| TEXAS INSTRUMENTS INCORPORATED
| Standard Linear and Logic Group
| IBIS Model of SN74LVCZ16245A
| 16-BIT BUS TRANSCEIVER WITH 3-STATE OUTPUTS
| This file contains package information for the following:
|  TSSOP 48-pin (DGG) package as [Component] LVCZ16245A_DGG
|  TVSOP 48-pin (DGV) package as [Component] LVCZ16245A_DGV
|  SSOP 48-pin (DL) package as [Component] LVCZ16245A_DL
| This device can be powered at the following Vccs:
|  2.7 volt Vcc
|  3.3 volt Vcc
| This file provides unique models under the [Model Selector] for each Vcc.
| For operation at a specific Vcc, select the appropriate model after each
| [Model Selector] keyword.
[IBIS Ver]   3.2
[Comment char]  |_char
[File Name]   sn74lvcz16245a.ibs
[File Rev]   1.1 | x_die
[Date]   March 01,2004
[Source]   Data created from TI-SPICE simulations at TI-SLL.
[Notes]   The following is an IBIS list for the LVCZ16245A.
   Please contact sllibis@ti.com with questions and
   comments concerning SLL IBIS models.
   - FILE REV HISTORY
   - 1.1 Release IBIS file on 03/02/04
   - Power clamp data deleted as there is no power-clamp diode.
[Disclaimer] Property of Texas Instruments Incorporated.  Unauthorized
   reproduction and/or distribution is strictly prohibited.
   This product is protected under copyright law.
   Created  2004, (C) Copyright  2004, Texas Instruments
   Incorporated, All Rights Reserved
   UNLESS THERE IS A SIGNED, WRITTEN AGREEMENT TO THE
   CONTRARY, TEXAS INSTRUMENTS (TI) IS PROVIDING THE IBIS
   MODELS  AND WITHOUT ANY WARRANTY, EXPRESSED OR
   IMPLIED.  TI assumes no liability for:
   1) the accuracy of the IBIS models provided to your
   company;
   2) the proper functioning of these IBIS Models in your
   design or for any resulting applications; or
   3) infringement of patents, copyrights or intellectual
   property rights resulting from your use of these IBIS
   models.
   TI provides IBIS Models as a service to our customers.
   You and your company shall not distribute, sell or give
   these models to anyone else without prior written
   permission from TI.
   TI reserves the right to make changes to our products or
   to discontinue any semiconductor product or service
   without notice, and advises our customers to obtain the
   latest version of relevant information to verify, before
   placing orders, that the information being relied on is
   current.
   Please be aware that your receipt and use of the IBIS
   information provided shall serve as acceptance of these
   terms and conditions.  If you do not accept these terms,
   you should return or destroy the IBIS models and any
   other accompanying information immediately.
| Component LVCZ16245A_DGG 48-pin TSSOP
[Component]   LVCZ16245A_DGG
[Manufacturer]   Texas Instruments, Inc.
[Package]
|   typ   min   max
R_pkg   4.400e-02   3.800e-02   5.100e-02
L_pkg   3.019e-09   2.486e-09   4.099e-09
C_pkg   5.070e-13   3.340e-13   8.090e-13
[Pin]   signal_name   model_name   R_pin   L_pin   C_pin
1   1DIR   LVCZ16245A_DIR   4.100e-02   4.017e-09   7.590e-13
2   1B1   LVCZ16245A_IO   4.200e-02   3.737e-09   7.920e-13
3   1B2   LVCZ16245A_IO   4.200e-02   3.480e-09   6.610e-13
4   GND   GND   3.800e-02   3.131e-09   5.750e-13
5   1B3   LVCZ16245A_IO   4.700e-02   3.122e-09   5.660e-13
6   1B4   LVCZ16245A_IO   4.300e-02   2.948e-09   5.040e-13
7   VCC   POWER   4.500e-02   2.845e-09   3.970e-13
8   1B5   LVCZ16245A_IO   4.900e-02   2.835e-09   3.940e-13
9   1B6   LVCZ16245A_IO   4.800e-02   2.715e-09   3.780e-13
10   GND   GND   5.000e-02   2.664e-09   3.630e-13
11   1B7   LVCZ16245A_IO   5.000e-02   2.585e-09   3.480e-13
12   1B8   LVCZ16245A_IO   4.900e-02   2.550e-09   3.370e-13
13   2B1   LVCZ16245A_IO   4.900e-02   2.541e-09   3.360e-13
14   2B2   LVCZ16245A_IO   5.000e-02   2.574e-09   3.480e-13
15   GND   GND   4.900e-02   2.618e-09   3.590e-13
16   2B3   LVCZ16245A_IO   4.600e-02   2.671e-09   3.750e-13
17   2B4   LVCZ16245A_IO   4.500e-02   2.754e-09   3.890e-13
18   VCC   POWER   4.400e-02   2.823e-09   4.500e-13
19   2B5   LVCZ16245A_IO   4.200e-02   2.968e-09   5.030e-13
20   2B6   LVCZ16245A_IO   5.100e-02   3.108e-09   5.350e-13
21   GND   GND   4.200e-02   3.175e-09   5.870e-13
22   2B7   LVCZ16245A_IO   4.100e-02   3.449e-09   6.780e-13
23   2B8   LVCZ16245A_IO   4.400e-02   3.766e-09   8.040e-13
24   2DIR   LVCZ16245A_DIR   4.300e-02   4.065e-09   7.610e-13
25   2OE   LVCZ16245A_NOE   4.100e-02   3.994e-09   7.570e-13
26   2A8   LVCZ16245A_IO   3.900e-02   3.649e-09   7.890e-13
27   2A7   LVCZ16245A_IO   3.800e-02   3.362e-09   6.600e-13
28   GND   GND   3.800e-02   3.082e-09   5.740e-13
29   2A6   LVCZ16245A_IO   4.400e-02   2.990e-09   5.220e-13
30   2A5   LVCZ16245A_IO   4.100e-02   2.917e-09   4.950e-13
31   VCC   POWER   4.300e-02   2.820e-09   4.480e-13
32   2A4   LVCZ16245A_IO   4.300e-02   2.699e-09   3.850e-13
33   2A3   LVCZ16245A_IO   4.500e-02   2.628e-09   3.720e-13
34   GND   GND   4.600e-02   2.556e-09   3.560e-13
35   2A2   LVCZ16245A_IO   4.600e-02   2.495e-09   3.440e-13
36   2A1   LVCZ16245A_IO   4.700e-02   2.487e-09   3.340e-13
37   1A8   LVCZ16245A_IO   4.700e-02   2.490e-09   3.350e-13
38   1A7   LVCZ16245A_IO   4.600e-02   2.486e-09   3.430e-13
39   GND   GND   4.500e-02   2.566e-09   3.560e-13
40   1A6   LVCZ16245A_IO   4.400e-02   2.639e-09   3.740e-13
41   1A5   LVCZ16245A_IO   4.300e-02   2.701e-09   3.860e-13
42   VCC   POWER   4.300e-02   2.817e-09   4.500e-13
43   1A4   LVCZ16245A_IO   4.100e-02   2.935e-09   5.010e-13
44   1A3   LVCZ16245A_IO   4.700e-02   3.035e-09   5.290e-13
45   GND   GND   4.300e-02   3.171e-09   5.890e-13
46   1A2   LVCZ16245A_IO   4.000e-02   3.415e-09   6.820e-13
47   1A1   LVCZ16245A_IO   4.300e-02   3.741e-09   8.090e-13
48   1OE   LVCZ16245A_NOE   4.400e-02   4.099e-09   7.640e-13
| Component LVCZ16245A_DGV 48-pin TVSOP
[Component]   LVCZ16245A_DGV
[Manufacturer]   Texas Instruments, Inc.
[Package]
|   typ   min   max
R_pkg   7.000e-02   4.900e-02   8.500e-02
L_pkg   3.013e-09   2.743e-09   3.408e-09
C_pkg   3.710e-13   2.940e-13   5.110e-13
[Pin]   signal_name   model_name   R_pin   L_pin   C_pin
1   1DIR   LVCZ16245A_DIR   4.900e-02   3.393e-09   4.970e-13
2   1B1   LVCZ16245A_IO   6.000e-02   3.250e-09   5.020e-13
3   1B2   LVCZ16245A_IO   7.700e-02   3.310e-09   4.510e-13
4   GND   GND   8.500e-02   3.299e-09   4.040e-13
5   1B3   LVCZ16245A_IO   8.300e-02   3.136e-09   3.600e-13
6   1B4   LVCZ16245A_IO   7.700e-02   3.019e-09   3.630e-13
7   VCC   POWER   6.500e-02   2.882e-09   3.490e-13
8   1B5   LVCZ16245A_IO   6.600e-02   2.829e-09   3.140e-13
9   1B6   LVCZ16245A_IO   6.700e-02   2.796e-09   3.140e-13
10   GND   GND   6.900e-02   2.754e-09   3.080e-13
11   1B7   LVCZ16245A_IO   7.000e-02   2.753e-09   3.010e-13
12   1B8   LVCZ16245A_IO   7.100e-02   2.745e-09   2.940e-13
13   2B1   LVCZ16245A_IO   7.000e-02   2.744e-09   2.940e-13
14   2B2   LVCZ16245A_IO   7.000e-02   2.754e-09   3.010e-13
15   GND   GND   6.900e-02   2.754e-09   3.080e-13
16   2B3   LVCZ16245A_IO   6.700e-02   2.796e-09   3.140e-13
17   2B4   LVCZ16245A_IO   6.600e-02   2.829e-09   3.140e-13
18   VCC   POWER   6.500e-02   2.883e-09   3.500e-13
19   2B5   LVCZ16245A_IO   7.500e-02   3.014e-09   3.630e-13
20   2B6   LVCZ16245A_IO   8.000e-02   3.128e-09   3.580e-13
21   GND   GND   8.400e-02   3.295e-09   4.030e-13
22   2B7   LVCZ16245A_IO   7.800e-02   3.311e-09   4.520e-13
23   2B8   LVCZ16245A_IO   6.200e-02   3.259e-09   5.010e-13
24   2DIR   LVCZ16245A_DIR   5.200e-02   3.404e-09   4.960e-13
25   2OE   LVCZ16245A_NOE   5.300e-02   3.397e-09   5.050e-13
26   2A8   LVCZ16245A_IO   6.200e-02   3.249e-09   5.110e-13
27   2A7   LVCZ16245A_IO   7.700e-02   3.308e-09   4.530e-13
28   GND   GND   8.200e-02   3.289e-09   4.030e-13
29   2A6   LVCZ16245A_IO   7.800e-02   3.121e-09   3.590e-13
30   2A5   LVCZ16245A_IO   7.400e-02   3.010e-09   3.630e-13
31   VCC   POWER   6.500e-02   2.883e-09   3.490e-13
32   2A4   LVCZ16245A_IO   6.700e-02   2.829e-09   3.140e-13
33   2A3   LVCZ16245A_IO   6.700e-02   2.795e-09   3.140e-13
34   GND   GND   6.900e-02   2.753e-09   3.070e-13
35   2A2   LVCZ16245A_IO   7.000e-02   2.753e-09   3.010e-13
36   2A1   LVCZ16245A_IO   7.000e-02   2.743e-09   2.940e-13
37   1A8   LVCZ16245A_IO   7.000e-02   2.743e-09   2.940e-13
38   1A7   LVCZ16245A_IO   7.000e-02   2.753e-09   3.010e-13
39   GND   GND   6.900e-02   2.754e-09   3.070e-13
40   1A6   LVCZ16245A_IO   6.800e-02   2.797e-09   3.140e-13
41   1A5   LVCZ16245A_IO   6.700e-02   2.830e-09   3.140e-13
42   VCC   POWER   6.400e-02   2.880e-09   3.490e-13
43   1A4   LVCZ16245A_IO   7.200e-02   3.004e-09   3.620e-13
44   1A3   LVCZ16245A_IO   7.800e-02   3.121e-09   3.590e-13
45   GND   GND   8.400e-02   3.296e-09   4.030e-13
46   1A2   LVCZ16245A_IO   7.700e-02   3.308e-09   4.510e-13
47   1A1   LVCZ16245A_IO   6.200e-02   3.258e-09   4.990e-13
48   1OE   LVCZ16245A_NOE   5.300e-02   3.408e-09   4.940e-13
| Component LVCZ16245A_DL 48-pin SSOP
[Component]   LVCZ16245A_DL
[Manufacturer]   Texas Instruments, Inc.
[Package]
|   typ   min   max
R_pkg   4.800e-02   3.800e-02   5.300e-02
L_pkg   6.046e-09   5.084e-09   7.968e-09
C_pkg   8.130e-13   5.690e-13   1.157e-12
[Pin]   signal_name   model_name   R_pin   L_pin   C_pin
1   1DIR   LVCZ16245A_DIR   4.600e-02   7.968e-09   1.017e-12
2   1B1   LVCZ16245A_IO   4.400e-02   7.299e-09   1.157e-12
3   1B2   LVCZ16245A_IO   4.300e-02   6.765e-09   1.058e-12
4   GND   GND   4.100e-02   6.269e-09   9.330e-13
5   1B3   LVCZ16245A_IO   3.800e-02   5.856e-09   8.290e-13
6   1B4   LVCZ16245A_IO   4.600e-02   5.802e-09   7.900e-13
7   VCC   POWER   5.000e-02   5.656e-09   7.380e-13
8   1B5   LVCZ16245A_IO   5.300e-02   5.500e-09   6.430e-13
9   1B6   LVCZ16245A_IO   5.200e-02   5.304e-09   6.060e-13
10   GND   GND   5.300e-02   5.189e-09   5.830e-13
11   1B7   LVCZ16245A_IO   5.100e-02   5.084e-09   5.690e-13
12   1B8   LVCZ16245A_IO   5.300e-02   5.862e-09   8.330e-13
13   2B1   LVCZ16245A_IO   5.300e-02   5.862e-09   8.330e-13
14   2B2   LVCZ16245A_IO   5.100e-02   5.084e-09   5.690e-13
15   GND   GND   5.300e-02   5.189e-09   5.830e-13
16   2B3   LVCZ16245A_IO   5.200e-02   5.304e-09   6.060e-13
17   2B4   LVCZ16245A_IO   5.300e-02   5.500e-09   6.430e-13
18   VCC   POWER   5.000e-02   5.656e-09   7.380e-13
19   2B5   LVCZ16245A_IO   4.600e-02   5.802e-09   7.900e-13
20   2B6   LVCZ16245A_IO   3.800e-02   5.856e-09   8.290e-13
21   GND   GND   4.100e-02   6.269e-09   9.330e-13
22   2B7   LVCZ16245A_IO   4.300e-02   6.765e-09   1.058e-12
23   2B8   LVCZ16245A_IO   4.400e-02   7.299e-09   1.157e-12
24   2DIR   LVCZ16245A_DIR   4.600e-02   7.968e-09   1.017e-12
25   2OE   LVCZ16245A_NOE   4.600e-02   7.968e-09   1.017e-12
26   2A8   LVCZ16245A_IO   4.400e-02   7.299e-09   1.157e-12
27   2A7   LVCZ16245A_IO   4.300e-02   6.765e-09   1.058e-12
28   GND   GND   4.100e-02   6.269e-09   9.330e-13
29   2A6   LVCZ16245A_IO   3.800e-02   5.856e-09   8.290e-13
30   2A5   LVCZ16245A_IO   4.600e-02   5.802e-09   7.900e-13
31   VCC   POWER   5.000e-02   5.656e-09   7.380e-13
32   2A4   LVCZ16245A_IO   5.300e-02   5.500e-09   6.430e-13
33   2A3   LVCZ16245A_IO   5.200e-02   5.304e-09   6.060e-13
34   GND   GND   5.300e-02   5.189e-09   5.830e-13
35   2A2   LVCZ16245A_IO   5.100e-02   5.084e-09   5.690e-13
36   2A1   LVCZ16245A_IO   5.300e-02   5.862e-09   8.330e-13
37   1A8   LVCZ16245A_IO   5.300e-02   5.862e-09   8.330e-13
38   1A7   LVCZ16245A_IO   5.100e-02   5.084e-09   5.690e-13
39   GND   GND   5.300e-02   5.189e-09   5.830e-13
40   1A6   LVCZ16245A_IO   5.200e-02   5.304e-09   6.060e-13
41   1A5   LVCZ16245A_IO   5.300e-02   5.500e-09   6.430e-13
42   VCC   POWER   5.000e-02   5.656e-09   7.380e-13
43   1A4   LVCZ16245A_IO   4.600e-02   5.802e-09   7.900e-13
44   1A3   LVCZ16245A_IO   3.800e-02   5.856e-09   8.290e-13
45   GND   GND   4.100e-02   6.269e-09   9.330e-13
46   1A2   LVCZ16245A_IO   4.300e-02   6.765e-09   1.058e-12
47   1A1   LVCZ16245A_IO   4.400e-02   7.299e-09   1.157e-12
48   1OE   LVCZ16245A_NOE   4.600e-02   7.967e-09   1.017e-12
| Model LVCZ16245A_DIR
[Model Selector]   LVCZ16245A_DIR
LVCZ16245A_DIR_27   2.7 volt Vcc
LVCZ16245A_DIR_33   3.3 volt Vcc
| Model LVCZ16245A_NOE
[Model Selector]   LVCZ16245A_NOE
LVCZ16245A_NOE_27   2.7 volt Vcc
LVCZ16245A_NOE_33   3.3 volt Vcc
| Model LVCZ16245A_IO
[Model Selector]   LVCZ16245A_IO
LVCZ16245A_IO_27   2.7 volt Vcc
LVCZ16245A_IO_33   3.3 volt Vcc
| Models and submodels in the file (6): LVCZ16245A_DIR_27 (Input), LVCZ16245A_DIR_33 (Input), LVCZ16245A_NOE_27 (Input), LVCZ16245A_NOE_33 (Input), LVCZ16245A_IO_27 (I/O), LVCZ16245A_IO_33 (I/O)
